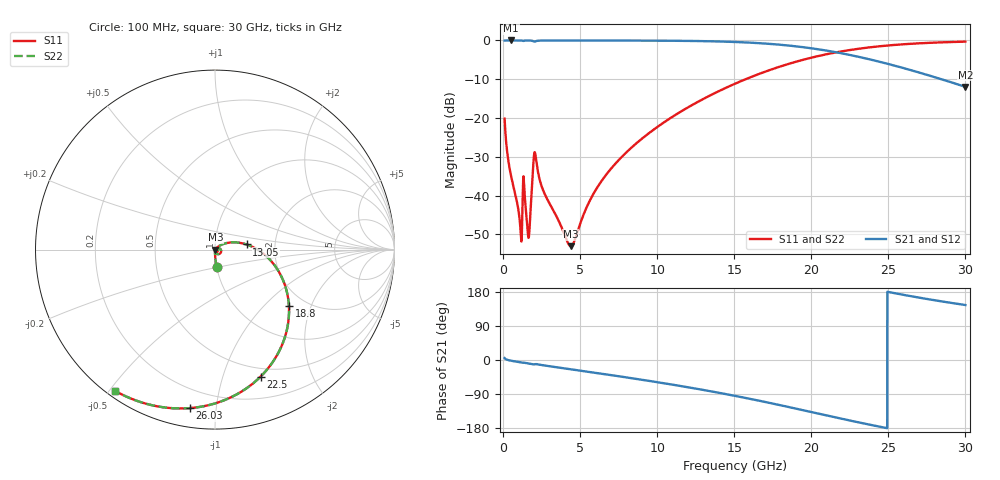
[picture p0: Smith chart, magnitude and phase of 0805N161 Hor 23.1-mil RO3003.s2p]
# GHz S MA R 50
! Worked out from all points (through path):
!   3201 points, 100 MHz to 30 GHz, reference 50 ohm
!   highest |S21| = -0.01 dB at 529.8 MHz (marker M1); lowest = -12.0 dB at 30 GHz (marker M2)
!   group delay of S21, straight-line fit = 20.9 ps
!   lowest |S11| = -53.0 dB at 4.398 GHz (marker M3), VSWR 1.00, Z = 50.2 - j0.0951 ohm
!   |S11| at or under -10 dB: start of sweep to 15.73 GHz
!   |S22| runs from -53.0 to -0.3 dB; largest |S21 - S12| = 0
!   S11 on the Smith chart (normalised r, x): 100 MHz: 1.00, -0.20; 13.05 GHz: 1.43, +0.08; 18.8 GHz: 1.65, -1.41; 22.5 GHz: 0.41, -1.34; 26.03 GHz: 0.10, -0.85; 30 GHz: 0.02, -0.52
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0.1  0.09818 -84.8  0.9949 5.1  0.9949 5.1  0.09818 -84.8
0.5298125  0.01753 -90.0  0.9992 -2.0  0.9992 -2.0  0.01753 -90.0
1.090437  0.00458 -79.8  0.9987 -5.9  0.9987 -5.9  0.00458 -79.8
1.398781  0.01062 -70.5  0.9951 -7.3  0.9951 -7.3  0.01062 -70.5
1.557625  0.004247 -63.9  0.9975 -8.6  0.9975 -8.6  0.004247 -63.9
1.641719  0.002888 -30.5  0.9972 -9.2  0.9972 -9.2  0.002888 -30.5
1.753844  0.004989 25.1  0.9958 -10.0  0.9958 -10.0  0.004989 25.1
1.96875  0.02669 13.3  0.9757 -11.7  0.9757 -11.7  0.02669 13.3
2.108906  0.03261 -50.2  0.9746 -10.6  0.9746 -10.6  0.03261 -50.2
2.6415  0.01118 -87.3  0.9966 -14.2  0.9966 -14.2  0.01118 -87.3
4.398125  0.002234 -25.1  0.9976 -24.5  0.9976 -24.5  0.002234 -25.1
5.089563  0.004853 32.9  0.9975 -28.5  0.9975 -28.5  0.004853 32.9
6.911594  0.02114 43.5  0.9969 -39.3  0.9969 -39.3  0.02114 43.5
10.06978  0.0782 28.5  0.9931 -58.9  0.9931 -58.9  0.0782 28.5
13.05044  0.1786 9.2  0.979 -79.4  0.979 -79.4  0.1786 9.2
15.05  0.2769 -5.7  0.9551 -94.6  0.9551 -94.6  0.2769 -5.7
18.79684  0.517 -37.2  0.8484 -126.4  0.8484 -126.4  0.517 -37.2
20.03956  0.6019 -48.3  0.7905 -137.6  0.7905 -137.6  0.6019 -48.3
22.49697  0.7518 -70.3  0.6503 -159.6  0.6503 -159.6  0.7518 -70.3
25.01978  0.8626 -91.2  0.496 179.3  0.496 179.3  0.8626 -91.2
26.02891  0.8939 -99.0  0.4379 171.6  0.4379 171.6  0.8939 -99.0
30  0.9644 -125.5  0.2523 145.1  0.2523 145.1  0.9644 -125.5
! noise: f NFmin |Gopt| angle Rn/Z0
0.1  0.0003888  0.8464  0.6414  0.0005381
3.417  0.006676  0.7179  19.13  0.004554
6.743  0.01006  0.6523  37.09  0.004971
10.06  0.01395  0.6396  53.95  0.005876
13.39  0.01839  0.6468  69.63  0.006802
16.7  0.02378  0.6672  84.1  0.007808
20.03  0.03081  0.698  97.67  0.008995
23.35  0.04046  0.7376  110.6  0.01047
26.67  0.05468  0.7844  123.3  0.01235
30  0.07719  0.8351  136  0.01459
